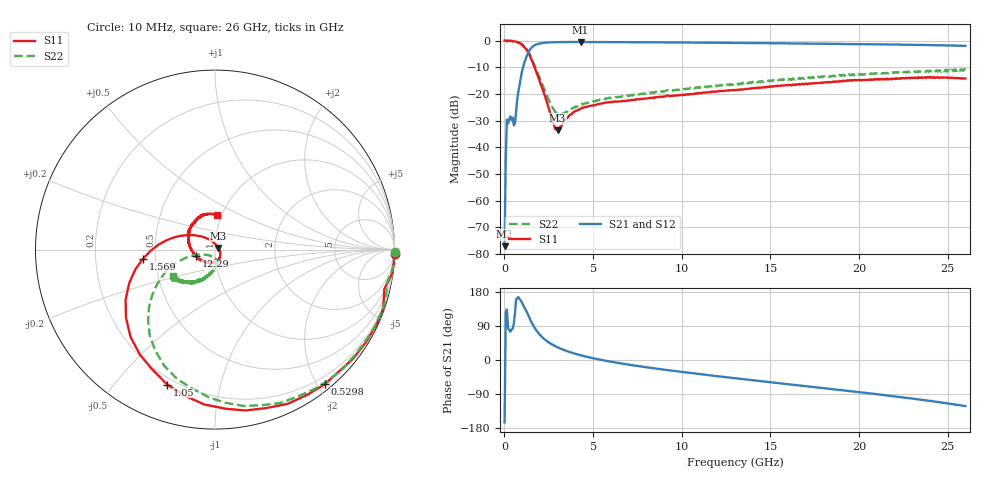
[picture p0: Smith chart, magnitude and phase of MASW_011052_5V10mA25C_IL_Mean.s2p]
! MA-COM, USA
! Part Number: MASW-011052
! Data: 29-03-2013
! Bias Condition:
!  Insertion Loss in ON stage Antenna (1) to RFin (2)
!  Forward Bias (series Diode and Shunt Diode) I = 10 mA
!  Reverse Bias Voltage V = -5V
!  Temp: 25C
!  VAR RecID: Mean
# HZ S DB R 50
! F n11x n11y n21x n21y n12x n12y n22x n22y
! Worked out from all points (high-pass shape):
!   401 points, 10 MHz to 26 GHz, reference 50 ohm
!   highest |S21| = -0.54 dB at 4.298 GHz (marker M1); lowest = -77.0 dB at 10 MHz (marker M2)
!   |S21| within 3 dB of the highest: 1.426 GHz to end of sweep
!   lowest |S11| = -33.6 dB at 2.999 GHz (marker M3), VSWR 1.04, Z = 51.9 + j0.985 ohm
!   |S11| at or under -10 dB: 1.698 GHz to end of sweep
!   |S22| runs from -27.7 to 0.0 dB; largest |S21 - S12| = 0.013
!   S11 on the Smith chart (normalised r, x): 10 MHz: -12, -89; 529.8 MHz: 0.09, -2.11; 1.05 GHz: 0.17, -0.69; 1.569 GHz: 0.42, -0.05; 12.29 GHz: 0.80, -0.06; 26 GHz: 0.95, +0.38
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1e7  0.03 -1.3  -77.00 -164.6  -77.98 -105.7  0.00 -0.8
2.0493e8  -0.06 -19.3  -31.05 85.4  -31.09 85.4  -0.06 -16.2
2.699e8  -0.07 -25.4  -29.40 78.4  -29.43 78.5  -0.09 -21.4
5.298e8  -0.28 -50.7  -31.79 95.4  -31.82 95.5  -0.23 -42.9
6.5975e8  -0.45 -64.8  -26.68 159.9  -26.70 160.1  -0.41 -54.6
7.897e8  -0.80 -79.2  -18.93 165.9  -18.95 166.2  -0.64 -66.8
1.0496e9  -1.97 -109.5  -10.12 146.0  -10.13 146.2  -1.69 -92.5
1.3095e9  -4.09 -142.6  -4.97 121.5  -4.97 121.7  -3.67 -120.4
1.5694e9  -7.85 -172.7  -2.42 95.7  -2.41 95.8  -7.25 -143.8
1.8293e9  -12.29 164.3  -1.41 76.2  -1.40 76.3  -11.43 -158.2
2.2192e9  -19.46 136.0  -0.87 56.5  -0.87 56.6  -17.74 -164.8
2.739e9  -30.61 82.9  -0.65 39.7  -0.65 39.7  -25.39 -146.0
2.9989e9  -33.62 27.1  -0.60 33.5  -0.61 33.5  -27.42 -125.9
3.7786e9  -27.58 -45.7  -0.55 19.5  -0.55 19.6  -25.56 -87.0
4.2984e9  -25.59 -62.0  -0.54 12.5  -0.55 12.5  -24.03 -81.0
4.3633e9  -25.17 -62.2  -0.55 11.7  -0.55 11.7  -23.76 -83.3
8.7167e9  -21.06 -127.0  -0.68 -23.7  -0.69 -23.6  -19.02 -92.4
1.229e10  -18.91 -160.8  -0.85 -44.3  -0.86 -44.0  -16.81 -104.6
1.3005e10  -18.57 -166.2  -0.90 -48.1  -0.89 -47.9  -16.55 -106.9
1.7358e10  -15.99 159.6  -1.16 -70.9  -1.20 -70.7  -13.70 -120.8
2.1712e10  -14.42 128.3  -1.47 -94.4  -1.47 -94.0  -11.98 -133.3
2.6e10  -14.21 87.0  -2.00 -121.7  -2.06 -121.2  -11.15 -147.6
